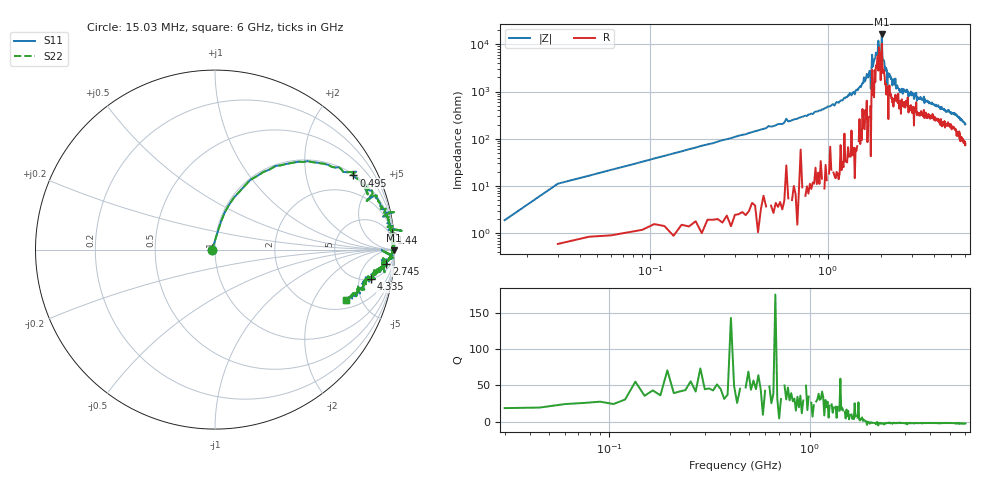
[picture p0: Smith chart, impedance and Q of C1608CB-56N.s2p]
!	Network	Analyzer	HP8753E.07.74:	Oct	30	2002	Serial	No.	JP38451487
!	Hewlett-Packard
!	7	Sep	2009	9:47:04
!	Frequency	S11	S21	S12	S22
#	HZ	S	RI	R	50
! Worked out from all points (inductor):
!   400 points, 15.03 MHz to 6 GHz, reference 50 ohm
!   read as one part in series: L = 58.2 nH near 45.03 MHz
!   highest |Z| = 16.1 kohm at 2.025 GHz (marker M1)
!   self-resonance near 1.92 GHz
!   S11 on the Smith chart (normalised r, x): 15.03 MHz: 0.97, -0.01; 495 MHz: 1.05, +3.70; 1.44 GHz: 2, +21; 2.745 GHz: 10, -19; 4.335 GHz: 4.89, -7.48; 6 GHz: 2.58, -3.73
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1.502992e7  -0.0172 -0.00477  1.02 0.00477  1.02 0.00477  -0.0172 -0.00477
3.002985e7  0.018 0.109  0.982 -0.109  0.982 -0.109  0.018 0.109
1.050295e8  0.137 0.324  0.863 -0.324  0.863 -0.324  0.137 0.324
4.950275e8  0.771 0.413  0.229 -0.413  0.229 -0.413  0.771 0.413
1.020025e9  0.952 0.196  0.0482 -0.196  0.0482 -0.196  0.952 0.196
1.440023e9  0.985 0.0936  0.0146 -0.0936  0.0146 -0.0936  0.985 0.0936
1.725021e9  0.999 0.0365  0.000733 -0.0365  0.000733 -0.0365  0.999 0.0365
1.755021e9  0.989 0.0863  0.0108 -0.0863  0.0108 -0.0863  0.989 0.0863
1.785021e9  0.992 0.0144  0.00815 -0.0144  0.00815 -0.0144  0.992 0.0144
1.800021e9  0.992 0.0285  0.00827 -0.0285  0.00827 -0.0285  0.992 0.0285
1.93502e9  0.998 -0.00812  0.00201 0.00812  0.00201 0.00812  0.998 -0.00812
2.01002e9  0.989 -0.00882  0.0115 0.00882  0.0115 0.00882  0.989 -0.00882
2.02502e9  0.996 -0.00473  0.00397 0.00473  0.00397 0.00473  0.996 -0.00473
2.04002e9  0.986 -0.0118  0.0142 0.0118  0.0142 0.0118  0.986 -0.0118
2.175019e9  0.928 -0.00351  0.0715 0.00351  0.0715 0.00351  0.928 -0.00351
2.190019e9  0.981 -0.0349  0.019 0.0349  0.019 0.0349  0.981 -0.0349
2.745016e9  0.954 -0.0785  0.0459 0.0785  0.0459 0.0785  0.954 -0.0785
3.015015e9  0.954 -0.0903  0.0459 0.0903  0.0459 0.0903  0.954 -0.0903
4.00501e9  0.895 -0.139  0.106 0.139  0.106 0.139  0.895 -0.139
4.335008e9  0.87 -0.165  0.13 0.165  0.13 0.165  0.87 -0.165
5.010005e9  0.834 -0.176  0.166 0.176  0.166 0.176  0.834 -0.176
6e9  0.732 -0.279  0.268 0.279  0.268 0.279  0.732 -0.279
